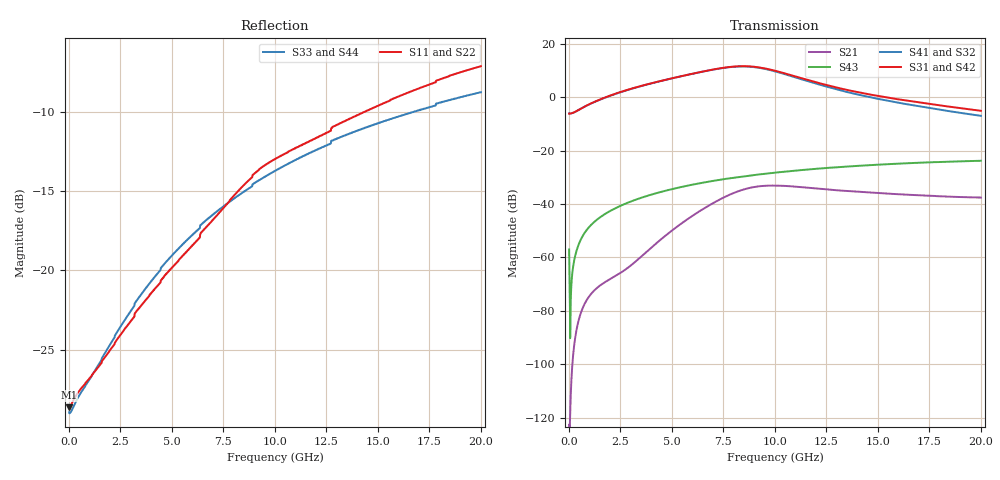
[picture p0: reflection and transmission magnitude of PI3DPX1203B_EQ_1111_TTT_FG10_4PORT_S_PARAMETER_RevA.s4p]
! NPort=4 DATA=2000 NOISE=0 GROUPDELAY=0 COMPLEX_DATAFORMAT=POLAR
! NumOfBlock=1 NumOfParam=0
! .MODEL Smodel S TSTONEFILE=PI3DPX1203B_EQ_1111_TTT_FG10_4PORT_S_PARAMETER_RevA.s4p TYPE=S
!  -- The above .MODEL line can be used for the S element in the netlist.
! The s parameter is extracted from the linear redriver, it is not bi-directional; only s(4,1)s(4,2) and s(3,1)s(3,2)
! should be the insertion loss
!Port definition:
!Port1 = input+
!Port2 = input-
!Port3 = output+
!Port4 = output-
# Hz S MA R  50
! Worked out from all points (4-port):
!   2000 points, 10 MHz to 20 GHz, reference 50 ohm
!   strongest paths, dB at 10 MHz, 5.01 GHz, 10.01 GHz, 15.01 GHz, 20 GHz:
!     S31: -6.2, 7.1, 9.9, 0.4, -5.1
!     S42: -6.2, 7.1, 9.9, 0.4, -5.1
!     S41: -6.2, 7.0, 9.6, -0.7, -7.0
!     S32: -6.2, 7.0, 9.6, -0.7, -7.0
!     S43: -57.1, -34.4, -28.3, -25.3, -23.8
!     S21: -122.7, -49.9, -33.1, -35.9, -37.6
!   lowest |S11| = -28.6 dB at 10 MHz (marker M1), VSWR 1.08, Z = 46.4 - j0.0306 ohm
!   |S11| at or under -10 dB: start of sweep to 14.39 GHz
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1e7  0.03701 -179.5  7.338e-07 10.7  0 0.0  0 0.0
     7.338e-07 10.7  0.03701 -179.5  0 0.0  0 0.0
     0.4917 0.0  0.4917 -180.0  0.03566 178.2  0.001403 -77.8
     0.4917 -180.0  0.4917 0.0  0.001403 -77.8  0.03566 178.2
2.97e9  0.06867 -127.8  0.0006877 148.8  1.169e-10 58.8  2.1e-09 108.4
        0.0006877 148.8  0.06867 -127.8  2.1e-09 108.4  1.169e-10 58.8
        1.417 6.2  1.405 -172.8  0.07383 -127.4  0.01097 78.1
        1.405 -172.8  1.417 6.2  0.01097 78.1  0.07383 -127.4
5.62e9  0.1127 -111.2  0.004761 156.4  9.637e-09 -123.1  9.176e-08 71.4
        0.00476 156.4  0.1127 -111.2  9.173e-08 71.4  9.638e-09 -123.1
        2.547 -37.2  2.545 144.1  0.1225 -117.5  0.02143 66.9
        2.545 144.1  2.547 -37.2  0.02143 66.9  0.1225 -117.5
8.03e9  0.1725 -104.8  0.01621 111.5  2.635e-07 155.3  7.482e-07 22.1
        0.0162 111.5  0.1725 -104.8  7.474e-07 22.1  2.635e-07 155.4
        3.74 -97.8  3.706 83.3  0.1684 -115.9  0.03112 54.8
        3.707 83.3  3.739 -97.8  0.03112 54.8  0.1684 -115.9
9.63e9  0.2166 -107.3  0.02201 67.3  9.744e-07 94.2  1.656e-06 -15.8
        0.02199 67.4  0.2166 -107.3  1.653e-06 -15.7  9.744e-07 94.3
        3.376 -149.0  3.3 32.0  0.1989 -116.1  0.03715 46.3
        3.301 32.0  3.375 -149.0  0.03715 46.3  0.1989 -116.1
1.19e10  0.2592 -109.5  0.01968 26.3  2.74e-06 29.2  3.384e-06 -44.5
         0.01967 26.4  0.2592 -109.5  3.384e-06 -44.4  2.741e-06 29.3
         1.941 161.7  1.833 -17.2  0.2375 -117.4  0.04514 34.7
         1.834 -17.2  1.94 161.7  0.04514 34.7  0.2375 -117.4
2e10  0.4394 -117.9  0.01312 -18.6  2.241e-05 -110.2  3.099e-05 -133.8
      0.01317 -18.6  0.4395 -117.9  3.106e-05 -133.8  2.243e-05 -110.2
      0.5548 72.3  0.4469 -96.0  0.3637 -123.9  0.06431 -7.1
      0.4466 -96.2  0.5552 72.4  0.06431 -7.1  0.3637 -123.9
